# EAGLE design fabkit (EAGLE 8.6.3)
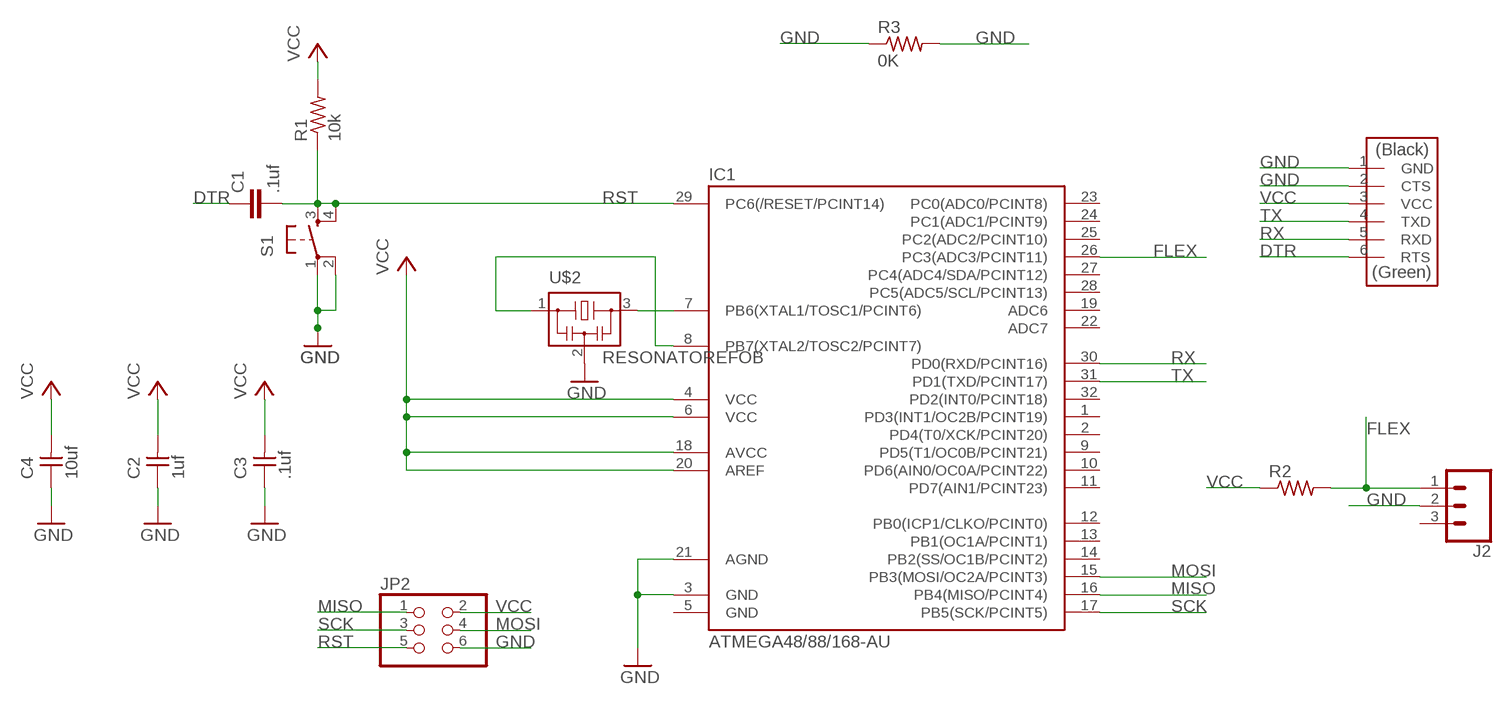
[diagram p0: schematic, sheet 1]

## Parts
C1  .1uf  C-EUC1206  [C1206]
C2  1uf  UNPOLARIZED_CAPACITOR1206  [1206]
C3  .1uf  UNPOLARIZED_CAPACITOR1206  [1206]
C4  10uf  UNPOLARIZED_CAPACITOR1206  [1206]
IC1  ATMEGA48/88/168-AU  [TQFP32-08]
J2  CONN_03LONGPADS  [1X03_LONGPADS]
JP2  PINHD-2X3-SMD  [2X03SMD]
R1  10k  RESISTOR1206  [1206]
R2  RES-US1206FAB  [R1206FAB]
R3  0K  RES-US1206FAB  [R1206FAB]
S1  6MM_SWITCH6MM_SWITCH  [6MM_SWITCH]
U$1  FTDI-SMD-HEADER  [1X06SMD]
U$2  RESONATOREFOB  [EFOBM]

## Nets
DTR: C1.1 U$1.6(RTS)
FLEX: IC1.26(PC3(ADC3/PCINT11)) J2.1 R2.2
GND: C2.1 C3.1 C4.1 IC1.3(GND) IC1.21(AGND) J2.2 JP2.6 R3.1 R3.2 S1.1(P) S1.2(P1) U$1.1(GND) U$1.2(CTS) U$2.2
MISO: IC1.16(PB4(MISO/PCINT4)) JP2.1
MOSI: IC1.15(PB3(MOSI/OC2A/PCINT3)) JP2.4
N$1: IC1.8(PB7(XTAL2/TOSC2/PCINT7)) U$2.1
N$2: IC1.7(PB6(XTAL1/TOSC1/PCINT6)) U$2.3
RST: C1.2 IC1.29(PC6(/RESET/PCINT14)) JP2.5 R1.1 S1.3(S) S1.4(S1)
RX: IC1.30(PD0(RXD/PCINT16)) U$1.5(RXD)
SCK: IC1.17(PB5(SCK/PCINT5)) JP2.3
TX: IC1.31(PD1(TXD/PCINT17)) U$1.4(TXD)
VCC: C2.2 C3.2 C4.2 IC1.4(VCC) IC1.6(VCC) IC1.18(AVCC) IC1.20(AREF) JP2.2 R1.2 R2.1 U$1.3(VCC)
Unconnected: IC1.1(PD3(INT1/OC2B/PCINT19)) IC1.2(PD4(T0/XCK/PCINT20)) IC1.9(PD5(T1/OC0B/PCINT21)) IC1.10(PD6(AIN0/OC0A/PCINT22)) IC1.11(PD7(AIN1/PCINT23)) IC1.12(PB0(ICP1/CLKO/PCINT0)) IC1.13(PB1(OC1A/PCINT1)) IC1.14(PB2(SS/OC1B/PCINT2)) IC1.19(ADC6) IC1.22(ADC7) IC1.23(PC0(ADC0/PCINT8)) IC1.24(PC1(ADC1/PCINT9)) IC1.25(PC2(ADC2/PCINT10)) IC1.27(PC4(ADC4/SDA/PCINT12)) IC1.28(PC5(ADC5/SCL/PCINT13)) IC1.32(PD2(INT0/PCINT18)) J2.3

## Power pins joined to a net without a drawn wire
GND: IC1.5(GND)

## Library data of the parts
C1 = rcl:C-EU: CAPACITOR, European symbol
C2-C4 = ng:UNPOLARIZED_CAPACITOR: unpolarized_capacitor
IC1 = atmega8:ATMEGA48/88/168
J2 = SparkFun-Connectors:CONN_03: Multi connection point. Often used as Generic Header-pin footprint for 0.1 inch spaced/style header connections On any of the 0.1 inch spaced packages, you can populate with these: Break Away Headers - Straight (PRT-00116) Break Away Male Headers - Right Angle (PRT-00553) Female Headers (PRT-00115)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
JP2 = fab:PINHD-2X3-SMD: PIN HEADER
R1 = ng:RESISTOR
R2 R3 = fab:RES-US: Resistor (US Symbol)
S1 = ng:6MM_SWITCH: OMRON SWITCH
U$1 = fab:FTDI-SMD-HEADER
U$2 = fab:RESONATOR

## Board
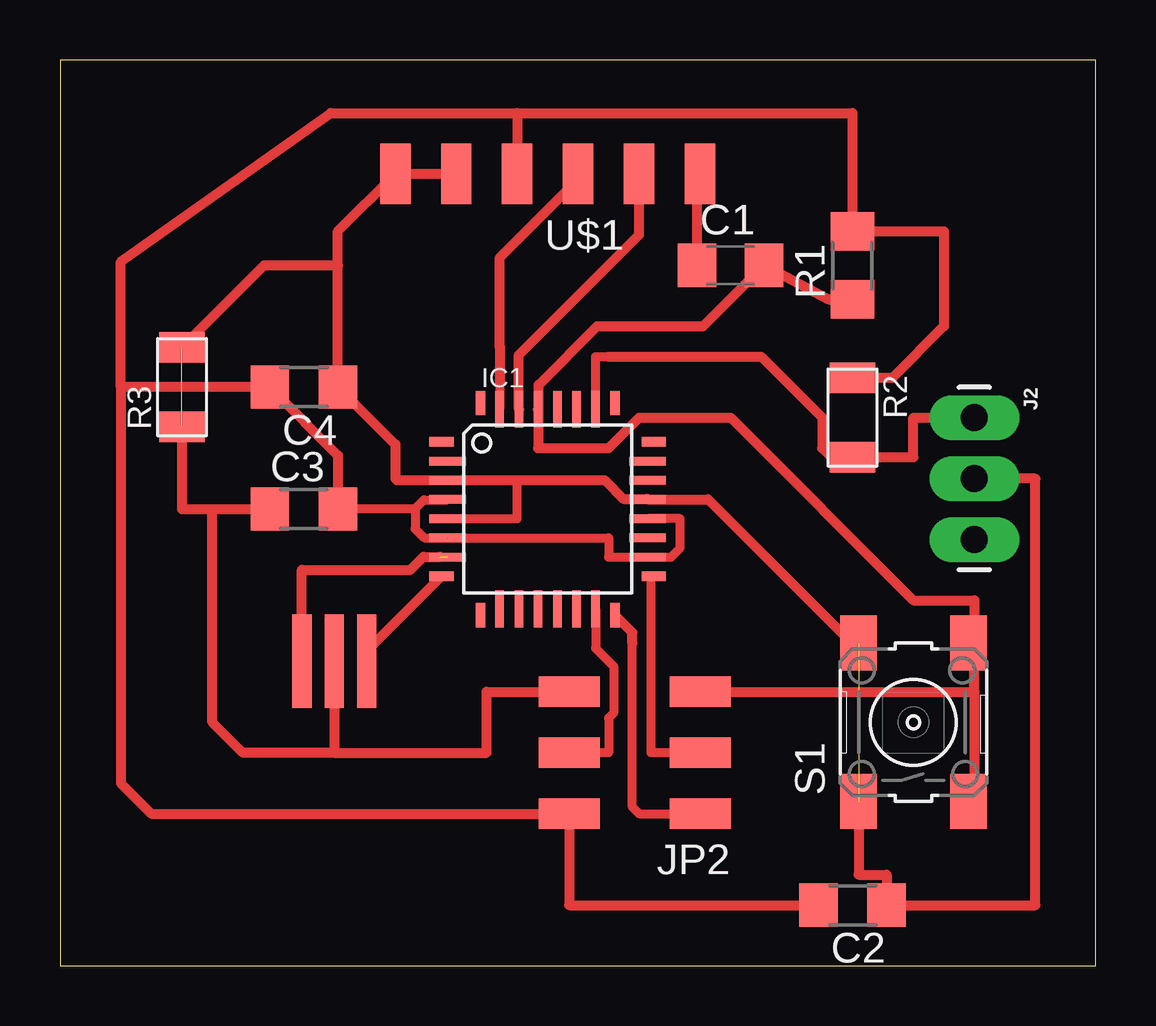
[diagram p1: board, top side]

Size 43.16 x 37.77 mm. Coordinates in mm from the lower left corner, seen from the top.
Outline: 0,0 43.16,0 43.16,37.77 0,37.77 0,0
Copper layers (1*16): Top 0.035mm / dielectric 1.5mm / Bottom 0.035mm
Design rules "default *": minimum track width 14mil, minimum drill 0.79mm, track to track 0.4mm, track to pad 0.4mm, pad to pad 0.4mm, via to via 0.4mm, smd to smd 6mil, copper to edge 40mil, drill to drill 6mil, minimum pad ring 10mil, minimum via ring 8mil, stop-mask expansion 4mil, vias tented up to drill 0mil, thermal gap 10mil

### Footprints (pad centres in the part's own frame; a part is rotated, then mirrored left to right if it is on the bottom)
C1206 = smd 1.6 x 1.8: 1 -1.4,0; 2 1.4,0
1206 = smd 1.6 x 1.803: 1 -1.422,0; 2 1.422,0
TQFP32-08 = smd 1.016 x 0.406: 1 -4.42,2.8; 8 -4.42,-2.8; 17 4.42,-2.8; 24 4.42,2.8 | smd 1.524 x 0.356: 2 -4.166,2; 3 -4.166,1.2; 4 -4.166,0.4; 5 -4.166,-0.4; 6 -4.166,-1.2; 7 -4.166,-2; 18 4.166,-2; 19 4.166,-1.2; 20 4.166,-0.4; 21 4.166,0.4; 22 4.166,1.2; 23 4.166,2 | smd 0.406 x 1.016: 9 -2.8,-4.42; 16 2.8,-4.42; 25 2.8,4.42; 32 -2.8,4.42 | smd 0.356 x 1.524: 10 -2,-4.166; 11 -1.2,-4.166; 12 -0.4,-4.166; 13 0.4,-4.166; 14 1.2,-4.166; 15 2,-4.166; 26 2,4.166; 27 1.2,4.166; 28 0.4,4.166; 29 -0.4,4.166; 30 -1.2,4.166; 31 -2,4.166
1X03_LONGPADS = drill 1.118 pad 1.88 long: 1 0,0; 2 2.54,0; 3 5.08,0
2X03SMD = smd 2.54 x 1.27: 1 -2.54,2.54; 2 2.92,2.54; 3 -2.54,0; 4 2.92,0; 5 -2.54,-2.54; 6 2.92,-2.54
R1206FAB = smd 1.27 x 1.905: 1 -1.651,0; 2 1.651,0
6MM_SWITCH = smd 2.286 x 1.524: 1 -3.302,2.286; 2 3.302,2.286; 3 -3.302,-2.286; 4 3.302,-2.286
1X06SMD = smd 2.54 x 1.27: 1 0,6.35; 2 0,3.81; 3 0,1.27; 4 0,-1.27; 5 0,-3.81; 6 0,-6.35
EFOBM = smd 0.8 x 3.9: 1 -1.35,0; 2 0,0; 3 1.35,0

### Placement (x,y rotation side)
C1  27.94,29.21 0 top
C2  33.02,2.54 180 top
C3  10.16,19.05 0 top
C4  10.16,24.13 180 top
IC1  20.32,19.05 0 top
J2  38.1,22.86 270 top
JP2  24.13,8.89 180 top
R1  33.02,29.21 90 top
R2  33.02,22.86 270 top
R3  5.08,24.13 90 top
S1  35.56,10.16 90 top
U$1  20.32,33.02 90 top
U$2  11.43,12.7 180 top

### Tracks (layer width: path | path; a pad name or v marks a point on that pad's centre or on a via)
DTR
  Top 0.406: U$1.6 26.54,33.02 C1.1
FLEX
  Top 0.381: IC1.26 22.32,25.4 22.86,25.4
  Top 0.406: 22.86,25.4 29.21,25.4 31.75,22.86 31.75,21.59 32.13,21.21 R2.2 35.56,21.21 35.56,22.86 J2.1
GND  (2 unrouted)
  Top 0.381: IC1.5 19.05,18.65 19.05,20.25
  Top 0.406: U$1.2 U$1.1 11.58,30.63 11.58,29.21 | U$2.2 11.43,8.89 | 11.43,8.89 7.62,8.89 6.35,10.16 6.35,19.05 | 11.43,8.89 17.78,8.89 17.78,11.43 JP2.6 | 33.27,6.25 S1.1 33.27,3.81 34.44,3.81 C2.1 40.64,2.54 40.64,20.32 J2.2 | S1.2 32.99,13.46 27,19.45 IC1.21 24.47,19.47 23.47,19.47 22.69,20.25 19.05,20.25 IC1.3 14.04,20.25 13.97,20.32 13.97,21.74 C4.1 11.58,29.21 | 6.35,19.05 C3.1 | R3.2 8.51,29.21 11.58,29.21 | R3.1 5.08,19.05 6.35,19.05
MISO
  Top 0.381: 23.85,13.46 23.85,6.63 24.13,6.35 JP2.1
  Top 0.406: 23.85,13.46 23.85,13.9 IC1.16
MOSI
  Top 0.381: JP2.4 22.86,8.89 22.86,10.34 23.07,10.55 23.07,12.49 22.32,13.24 IC1.15
N$1
  Top 0.406: U$2.1 12.78,13.13 IC1.8
N$2  (1 unrouted)
  Top 0.406: U$2.3 10.08,16.51 14.6,16.51 15.14,17.06 15.83,17.06
RST
  Top 0.406: R1.1 32.03,27.79 C1.2 26.8,26.67 22.38,26.67 19.94,24.23 19.94,23.23 IC1.29 19.92,21.59 22.86,21.59 24.13,22.86 27.94,22.86 35.56,15.24 38.1,15.24 38.1,13.46 | JP2.5 38.1,11.43 | 38.1,11.43 38.1,13.46 | 38.1,13.46 S1.4 | 38.1,11.43 38.1,6.86 S1.3
RX
  Top 0.406: IC1.30 19.12,25.47 24.13,30.48 U$1.5
SCK
  Top 0.381: JP2.3 24.63,8.89 24.63,16.25 IC1.17
TX
  Top 0.381: 18.31,24.24 18.32,24.23 IC1.31
  Top 0.406: 18.31,24.24 18.31,25.8 18.33,25.82 18.33,29.54 21.59,32.8 U$1.4
VCC  (1 unrouted)
  Top 0.381: IC1.20 25.84,18.65 25.84,17.43 25.46,17.05 IC1.18 22.86,17.05 22.86,17.85 IC1.6 15.18,17.85 14.8,18.23 14.8,19.07 | C3.2 14.78,19.05 14.8,19.07 | IC1.4 16.14,19.43 15.16,19.43 14.8,19.07
  Top 0.406: 2.54,24.13 2.54,29.36 11.28,35.56 19.05,35.56 | 19.05,35.56 U$1.3 | 19.05,35.56 33.02,35.56 R1.2 36.83,30.63 36.83,26.67 34.67,24.51 R2.1 | C2.2 21.21,2.54 JP2.2 3.81,6.35 2.54,7.62 2.54,24.13 | 2.54,24.13 C4.2 11.58,21.29 C3.2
